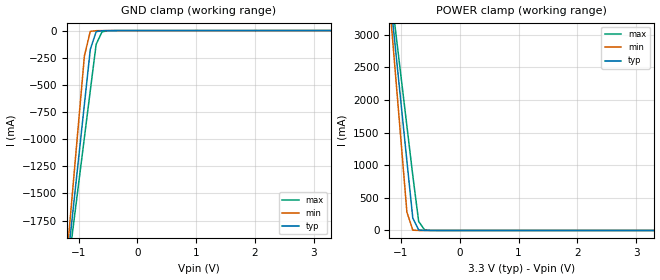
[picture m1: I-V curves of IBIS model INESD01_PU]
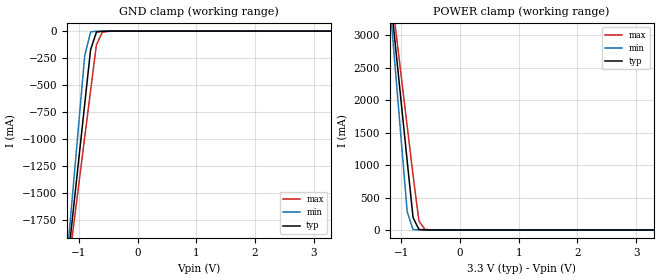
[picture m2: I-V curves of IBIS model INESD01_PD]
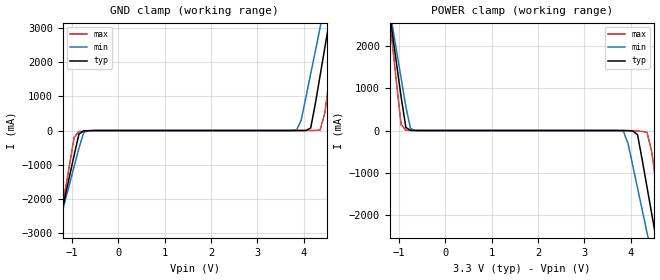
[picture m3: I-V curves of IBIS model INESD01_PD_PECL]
|   This file is an IBIS representation of the   |
|   Integrated Device Technology, Inc.   |
|   ICS8533-01   |
|   LOW SKEW, 1-TO-4 DIFFERENTIAL-TO-3.3V LVPECL FANOUT BUFFER   |
[IBIS Ver]   4.1
[File name]   8533_01_3v3.ibs
[File Rev]   2.0
[Date]   2 Feb 2009 | Last modified
|   Dec 11 2000 | Generated
[Source]   Originated at Integrated Devices Technology, Inc.
[Disclaimer]
IDT hereby grants the user of this IBIS model a non-exclusive,
nontransferable license to use this IBIS model under the following terms.
Before using this IBIS model, the user should read this license.
If the user does not accept these terms,  the IBIS model should be
returned to IDT within 30 days.
   The user is granted this license only to use the IBIS model and
is not granted rights to sell, load, rent, lease or license the IBIS
model in whole or in part, or in modified form to anyone other than
user. User may modify the IBIS model to suit its specific
applications but rights to derivative works and such modifications
shall belong to IDT.
   This IBIS model is provided on an "AS IS" basis and IDT makes
absolutely no warranty with respect to the information contained
herein. IDT DISCLAIMS AND CUSTOMER WAIVES ALL WARRANTIES, EXPRESS
OR IMPLIED, INCLUDING WARRANTIES OF MERCHANTABILITY OR FITNESS FOR
A PARTICULAR PURPOSE. The entire risk as to quality and performance
is with the Customer. ACCORDINGLY, IN NO EVENT SHALL THE COMPANY BE
LIABLE FOR ANY DAMAGES, WHETHER IN CONTRACT OR TORT,INCLUDING ANY
LOST PROFITS OR OTHER INCIDENTAL, CONSEQUENTIAL, EXEMPLARY, OR
PUNITIVE DAMAGES ARISING OUT OF THE USE OR APPLICATION OF THE IBIS
model provided in this package. Further, IDT reserves the right to
make changes without notice to any product herein to improve
reliability, function, or design. IDT does not convey any license
under patent rights or any other intellectual property rights,
including those of third parties.
   IDT is not obligated to provide maintenance or support
for the licensed IBIS model.
[Copyright]   Copyright 2005 by Integrated Device Technology, Inc.
[Component]   8533-01
[Manufacturer] Integrated Devices Technology, Inc.
[Package]
|TSSOP 20 Lead
|   typ   min   max
R_pkg   51.85m   41.1m   62.6m
L_pkg   1.568nH   0.734nH   2.401nH
C_pkg   0.221pF   0.068pF   0.373pF
[Pin]   signal_name   model_name   R_pin   L_pin   C_pin
1   VEE   GND   62.6m   2.401n   0.373p
2   CLK_EN   INESD01_PU   57.23m   1.985n   0.297p
3   CLK_SEL   INESD01_PD   51.85m   1.568n   0.221p
4   CLK   INESD01_PD_PECL   46.78m   1.151n   0.145p
5   nCLK   INESD01_PU_PECL   41.1m   0.734n   0.068p
6   PCLK   INESD01_PD_PECL   41.1m   0.734n   0.068p
7   nPCLK   INESD01_PU_PECL   46.78m   1.151n   0.145p
8   NC   NC   51.85m   1.568n   0.221p
9   NC   NC   57.23m   1.985n   0.297p
10   VCC   POWER   62.6m   2.401n   0.373p
11   nQ3   ONF01_PECL01ALT   62.6m   2.401n   0.373p
12   Q3   ONF01_PECL01ALT   57.23m   1.985n   0.297p
13   VCC   POWER   51.85m   1.568n   0.221p
14   nQ2   ONF01_PECL01ALT   46.78m   1.151n   0.145p
15   Q2   ONF01_PECL01ALT   41.1m   0.734n   0.068p
16   nQ1   ONF01_PECL01ALT   41.1m   0.734n   0.068p
17   Q1   ONF01_PECL01ALT   46.78m   1.151n   0.145p
18   VCC   POWER   51.85m   1.568n   0.221p
19   nQ0   ONF01_PECL01ALT   57.23m   1.985n   0.297p
20   Q0   ONF01_PECL01ALT   62.6m   2.401n   0.373p
[Diff Pin]  inv_pin  vdiff tdelay_typ tdelay_min  tdelay_max
12   11   NA   0  0  0
15   14   NA   0  0  0
17   16   NA   0  0  0
20   19   NA   0  0  0
| Models and submodels in the file (5): INESD01_PU (Input), INESD01_PD (Input), INESD01_PD_PECL (Input), INESD01_PU_PECL (Input), ONF01_PECL01ALT (Output_ECL)
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[Model]   INESD01_PU
Model_type   Input
Polarity   Non-Inverting
Vinl = 0.8V
Vinh = 2.0V
|   typ   min   max
C_comp   2pF   1.5pF   2.5pF
|   typ   min   max
[Voltage range]  3.3V   3.15V   3.45V
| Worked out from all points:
|   GND clamp passes 1 mA (typ) near -0.55 V on its own axis
|   POWER clamp passes 1 mA (typ) near -0.61 V on its own axis
[GND_clamp]
|Voltage   I(typ)   I(min)   I(max)
-3.3V     -12.83A    -15.14A    -11.37A
-1.2V     -2.195A    -2.092A    -2.281A
-1.1V     -1.689A    -1.472A    -1.849A
-900mV    -678.5mA   -232.7mA   -984.8mA
-800mV    -174mA     -7.237mA   -553.3mA
-700mV    -9.767mA   -1.114mA   -126.1mA
-600mV    -1.7mA     -240.1uA   -11.15mA
-300mV    -81.66uA   -67.79uA   -163.4uA
3.3V      1.866nA    1.113pA    239.1nA
[POWER_clamp]
|Voltage   I(typ)   I(min)   I(max)
-3.3V     22.38A     26.45A     19.82A
-1.2V     3.723A     3.545A     3.874A
-1.1V     2.836A     2.457A     3.116A
-1V       1.949A     1.369A     2.358A
-900mV    1.063A     281mA      1.601A
-800mV    191.5mA    5.012mA    843.9mA
-700mV    8.032mA    142.2uA    138.3mA
-600mV    607uA      17.63uA    10.62mA
-400mV    16.32uA    7.545uA    335.9uA
3.3V      -71.13uA   -62.11uA   -78.26uA
[Model]   INESD01_PD
Model_type   Input
Polarity   Non-Inverting
Vinl = 0.80V
Vinh = 2.0V
|   typ   min   max
C_comp   2pF   1.5pF   2.5pF
|   typ   min   max
[Voltage range]  3.3V   3.15V   3.45V
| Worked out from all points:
|   GND clamp passes 1 mA (typ) near -0.55 V on its own axis
|   POWER clamp passes 1 mA (typ) near -0.60 V on its own axis
[GND_clamp]
|Voltage I(typ)   I(min)   I(max)
-3.3V     -12.83A    -15.14A    -11.37A
-1.2V     -2.195A    -2.092A    -2.281A
-1.1V     -1.689A    -1.472A    -1.849A
-900mV    -678.5mA   -232.6mA   -984.8mA
-800mV    -173.9mA   -7.175mA   -553.2mA
-700mV    -9.696mA   -1.052mA   -126mA
-600mV    -1.629mA   -178uA     -11.07mA
-300mV    -10.53uA   -5.678uA   -86.08uA
3.3V      71.13uA    62.11uA    77.58uA
[POWER_clamp]
|Voltage   I(typ)   I(min)   I(max)
-3.3V     22.38A     26.45A     19.82A
-1.2V     3.723A     3.545A     3.874A
-1.1V     2.836A     2.457A     3.116A
-1V       1.949A     1.369A     2.358A
-900mV    1.063A     281.1mA    1.601A
-800mV    191.6mA    5.074mA    844mA
-700mV    8.104mA    204.3uA    138.4mA
-600mV    678.1uA    79.74uA    10.7mA
-400mV    87.44uA    69.65uA    413.2uA
3.3V      -3.041nA   -425fA     -919.9nA
[Model]   INESD01_PD_PECL
Model_type  Input
Polarity   Non-Inverting
Vinl = 0.8V
Vinh = 2.0V
|   typ   min   max
C_comp   2pF   1.5pF   2.5pF
|   typ   min   max
[Voltage range]  3.3V   3.15V   3.45V
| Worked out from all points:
|   GND clamp passes 1 mA (typ) near -0.55 V on its own axis
|   POWER clamp passes 1 mA (typ) near -0.66 V on its own axis
[GND_clamp]
|Voltage   I(typ)   I(min)   I(max)
-2.586V   -10.86A    -9.487A    -13.15A
-1.361V   -3.24A     -3.145A    -3.432A
-1.259V   -2.606A    -2.617A    -2.622A
-952.6mV  -705.3mA   -1.038A    -192.4mA
-850.5mV  -99.9mA    -513.5mA   -31.23mA
-646.4mV  -3.788mA   -3.549mA   -8.297mA
3.844V    129.1uA    13.13mA    71.12uA
4.151V    73.33mA    1.652A     864.7uA
4.355V    1.607A     3.003A     15.44mA
4.559V    3.233A     4.356A     1.553A
4.763V    4.861A     5.711A     3.635A
5.375V    9.757A     9.783A     9.893A
[POWER_clamp]
|Voltage   I(typ)   I(min)   I(max)
-2.177V   10.57A     9.364A     12.62A
-1.157V   2.42A      2.586A     2.194A
-952.6mV  795.8mA    1.237A     137.8mA
-850.5mV  73.33mA    563.2mA    8.145mA
-646.4mV  535.8uA    2.004mA    431.2uA
3.844V    -826.3uA   -18.14mA   -47.07uA
4.151V    -99.9mA    -1.362A    -11.82mA
4.355V    -1.338A    -2.415A    -41.71mA
4.559V    -2.606A    -3.47A     -1.312A
4.661V    -3.24A     -3.998A    -2.123A
4.763V    -3.875A    -4.526A    -2.933A
5.579V    -8.954A    -8.756A    -9.414A
